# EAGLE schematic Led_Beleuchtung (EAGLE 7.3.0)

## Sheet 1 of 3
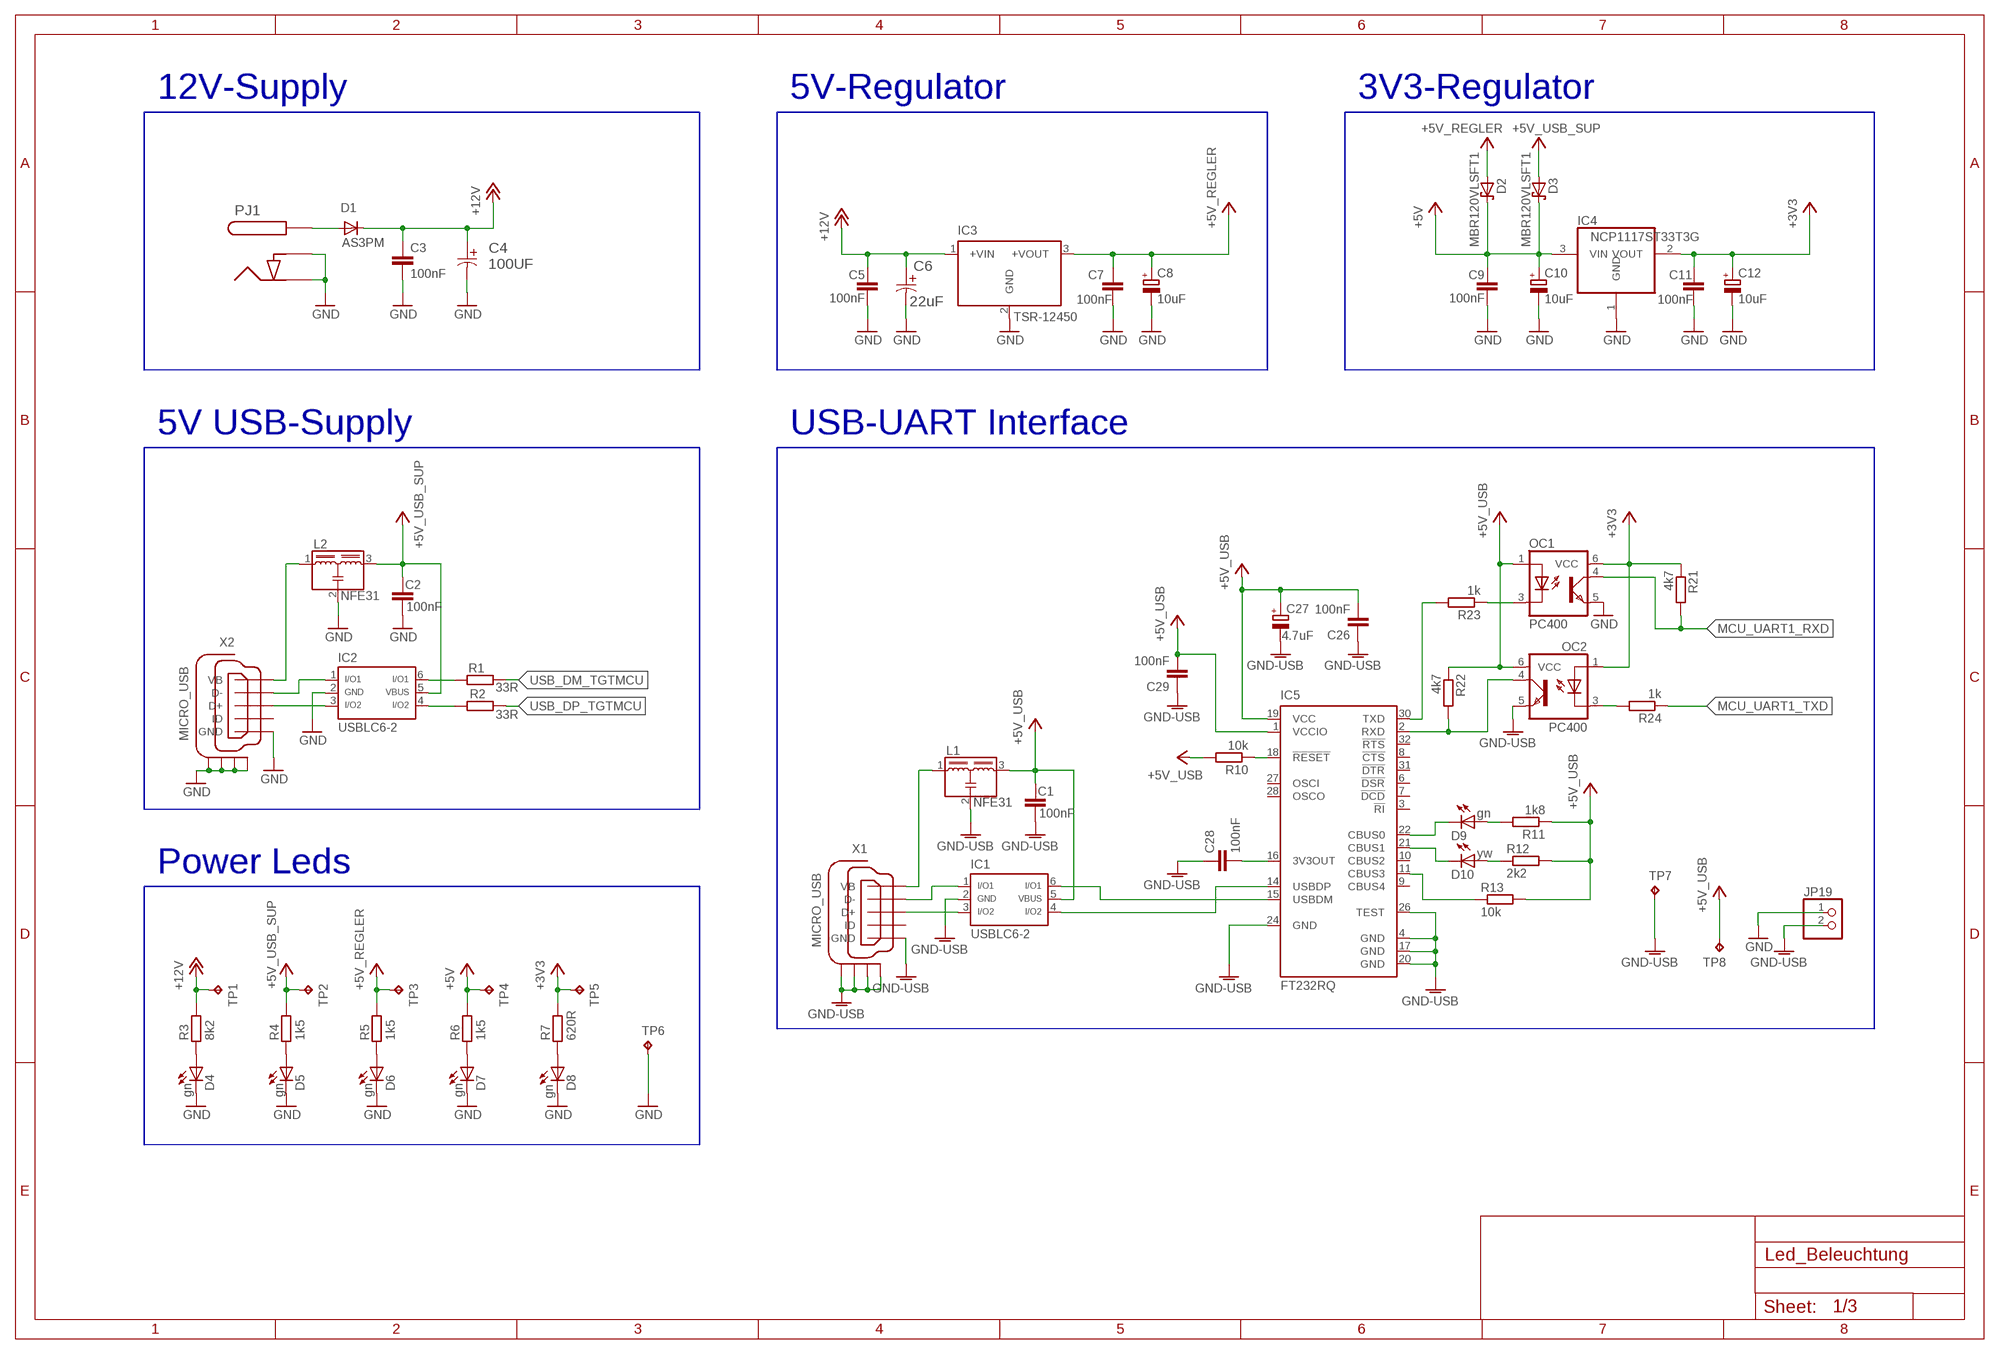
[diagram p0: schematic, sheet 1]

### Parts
C1  100nF  C-EUC0603K  [C0603K]
C2  100nF  C-EUC0603K  [C0603K]
C3  100nF  C-EUC0603K  [C0603K]
C4  100UF  EEE-FTH101XAP-CASE-D8  [CAPAE660X800N]
C5  100nF  C-EUC0603K  [C0603K]
C6  22uF  EEE--CASE-D  [CAPAE660X610N]
C7  100nF  C-EUC0603K  [C0603K]
C8  10uF  CPOL_EU0805  [SMC_P]
C9  100nF  C-EUC0603K  [C0603K]
C10  10uF  CPOL_EU0805  [SMC_P]
C11  100nF  C-EUC0603K  [C0603K]
C12  10uF  CPOL_EU0805  [SMC_P]
C26  100nF  C-EUC0603K  [C0603K]
C27  4.7uF  CPOL_EU0805  [SMC_P]
C28  100nF  C-EUC0603K  [C0603K]
C29  100nF  C-EUC0603  [C0603]
D1  AS3PM  [TO-277A]
D2  MBR120VLSFT1  [SOD-123]
D3  MBR120VLSFT1  [SOD-123]
D4  gn  LEDCHIP-LED0603  [CHIP-LED0603]
D5  gn  LEDCHIP-LED0603  [CHIP-LED0603]
D6  gn  LEDCHIP-LED0603  [CHIP-LED0603]
D7  gn  LEDCHIP-LED0603  [CHIP-LED0603]
D8  gn  LEDCHIP-LED0603  [CHIP-LED0603]
D9  gn  LEDCHIP-LED0603  [CHIP-LED0603]
D10  yw  LEDCHIP-LED0603  [CHIP-LED0603]
IC1  USBLC6-2  [SOT-23-6L]
IC2  USBLC6-2  [SOT-23-6L]
IC3  TSR-12450  [TSR-1]
IC4  NCP1117ST33T3G  REG1117  [SOT223]
IC5  FT232RQ  [QFN32]
JP19  PINHD-1X2  [1X02]
L1  NFE31  EMIFIL  [EMIFILTER]
L2  NFE31  EMIFIL  [EMIFILTER]
OC1  PC400  [PC400]
OC2  PC400  [PC400]
PJ1  PJ-002AH-SMT-TR  [PJ-002AH-SMT-TR]
R1  33R  R-EU_R0603  [R0603]
R2  33R  R-EU_R0603  [R0603]
R3  8k2  R-EU_R0603  [R0603]
R4  1k5  R-EU_R0603  [R0603]
R5  1k5  R-EU_R0603  [R0603]
R6  1k5  R-EU_R0603  [R0603]
R7  620R  R-EU_R0603  [R0603]
R10  10k  R-EU_R0603  [R0603]
R11  1k8  R-EU_R0603  [R0603]
R12  2k2  R-EU_R0603  [R0603]
R13  10k  R-EU_R0603  [R0603]
R21  4k7  R-EU_R0603  [R0603]
R22  4k7  R-EU_R0603  [R0603]
R23  1k  R-EU_R0603  [R0603]
R24  1k  R-EU_R0603  [R0603]
TP1  +12V  TPTP08R  [TP08R]
TP2  +5V_USB  TPTP08R  [TP08R]
TP3  +5V_Reg  TPTP08R  [TP08R]
TP4  +5V  TPTP08R  [TP08R]
TP5  +3V3  TPTP08R  [TP08R]
TP6  GND  TPTP08R  [TP08R]
TP7  GND  TPTP08R  [TP08R]
TP8  +5V  TPTP08R  [TP08R]
X1  MICRO_USB  [MICRO-USB]
X2  MICRO_USB  [MICRO-USB]

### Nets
3V3OUT_FT232: C28.2 IC5.16(3V3OUT)
+3V3: C11.2 C12.+ IC4.2(VOUT) OC1.6(VCC) OC2.1(A) R7.2 R21.1 TP5.TP ; also sheet 2
+5V: C9.2 C10.+ D2.C D3.C IC4.3(VIN) R6.2 TP4.TP ; also sheet 2
+5V_REGLER: C7.2 C8.+ D2.A IC3.3(+VOUT) R5.2 TP3.TP
+5V_USB: C1.2 C26.2 C27.+ C29.2 IC1.5 IC5.1(VCCIO) IC5.19(VCC) L1.3 OC1.1(A) OC2.6(VCC) R10.2 R11.1 R12.2 R13.2 R22.1 TP8.TP
+5V_USB_SUP: C2.2 D3.A IC2.5 L2.3 R4.2 TP2.TP
+12V: C3.2 C4.1 C5.2 C6.1 D1.C IC3.1(+VIN) R3.2 TP1.TP ; also sheet 3
GND: C2.1 C3.1 C4.2 C5.1 C6.2 C7.1 C8.- C9.1 C10.- C11.1 C12.- D4.C D5.C D6.C D7.C D8.C IC2.2 IC3.2(GND) IC4.1(GND) JP19.1 L2.2 OC1.5(EMI) PJ1.2 PJ1.3 TP6.TP X2.5(GND) X2.GND1(S1) X2.GND2(S2) X2.GND3(S3) X2.GND4(S4) ; also sheet 2,3
GND-USB: C1.1 C26.1 C27.- C28.1 C29.1 IC1.2 IC5.4(GND) IC5.17(GND) IC5.20(GND) IC5.24(GND) IC5.26(TEST) JP19.2 L1.2 OC2.5(EMI) TP7.TP X1.5(GND) X1.GND1(S1) X1.GND2(S2) X1.GND3(S3) X1.GND4(S4)
MCU_UART1_RXD: OC1.4(COL) R21.2 ; also sheet 2
MCU_UART1_TXD: R24.1 ; also sheet 2
N$3: IC5.18(!RESET) R10.1
N$9: D9.C IC5.22(CBUS0)
N$13: L1.1 X1.1(VB)
N$14: IC1.1 X1.2(D-)
N$15: IC1.3 X1.3(D+)
N$16: D4.A R3.1
N$17: L2.1 X2.1(VB)
N$18: D5.A R4.1
N$19: D10.C IC5.21(CBUS1)
N$21: D10.A R12.1
N$22: D9.A R11.2
N$23: IC5.11(CBUS3) R13.1
N$26: IC2.1 X2.2(D-)
N$27: IC2.3 X2.3(D+)
N$48: IC2.4 R2.1
N$49: IC2.6 R1.1
N$61: D6.A R5.1
N$86: D1.A1(A) D1.A2(A) PJ1.1.1 PJ1.1.2
N$88: D7.A R6.1
N$90: D8.A R7.1
N$91: OC1.3(C) R23.1
N$93: OC2.3(C) R24.2
N$95: IC5.30(TXD) R23.2
N$97: IC5.2(RXD) OC2.4(COL) R22.2
USB_DM_FT232: IC1.6 IC5.15(USBDM)
USB_DM_TGTMCU: R1.2 ; also sheet 2
USB_DP_FT232: IC1.4 IC5.14(USBDP)
USB_DP_TGTMCU: R2.2 ; also sheet 2
Unconnected: IC5.3(!RI) IC5.6(!DSR) IC5.7(!DCD) IC5.8(!CTS) IC5.9(CBUS4) IC5.10(CBUS2) IC5.27(OSCI) IC5.28(OSCO) IC5.31(!DTR) IC5.32(!RTS) X1.4(ID) X2.4(ID)

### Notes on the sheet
- 12V-Supply | 5V-Regulator | 3V3-Regulator
- 5V USB-Supply | USB-UART Interface
- Power Leds
- http://www.molex.com/pdm_docs/sd/5031821853_sd.pdf 
  http://pinouts.ru/Memory/sdcard_pinout.shtml 
  http://www.interfacebus.com/Secure_Digital_Card_Pinout.html 
  https://en.wikipedia.org/wiki/Secure_Digital

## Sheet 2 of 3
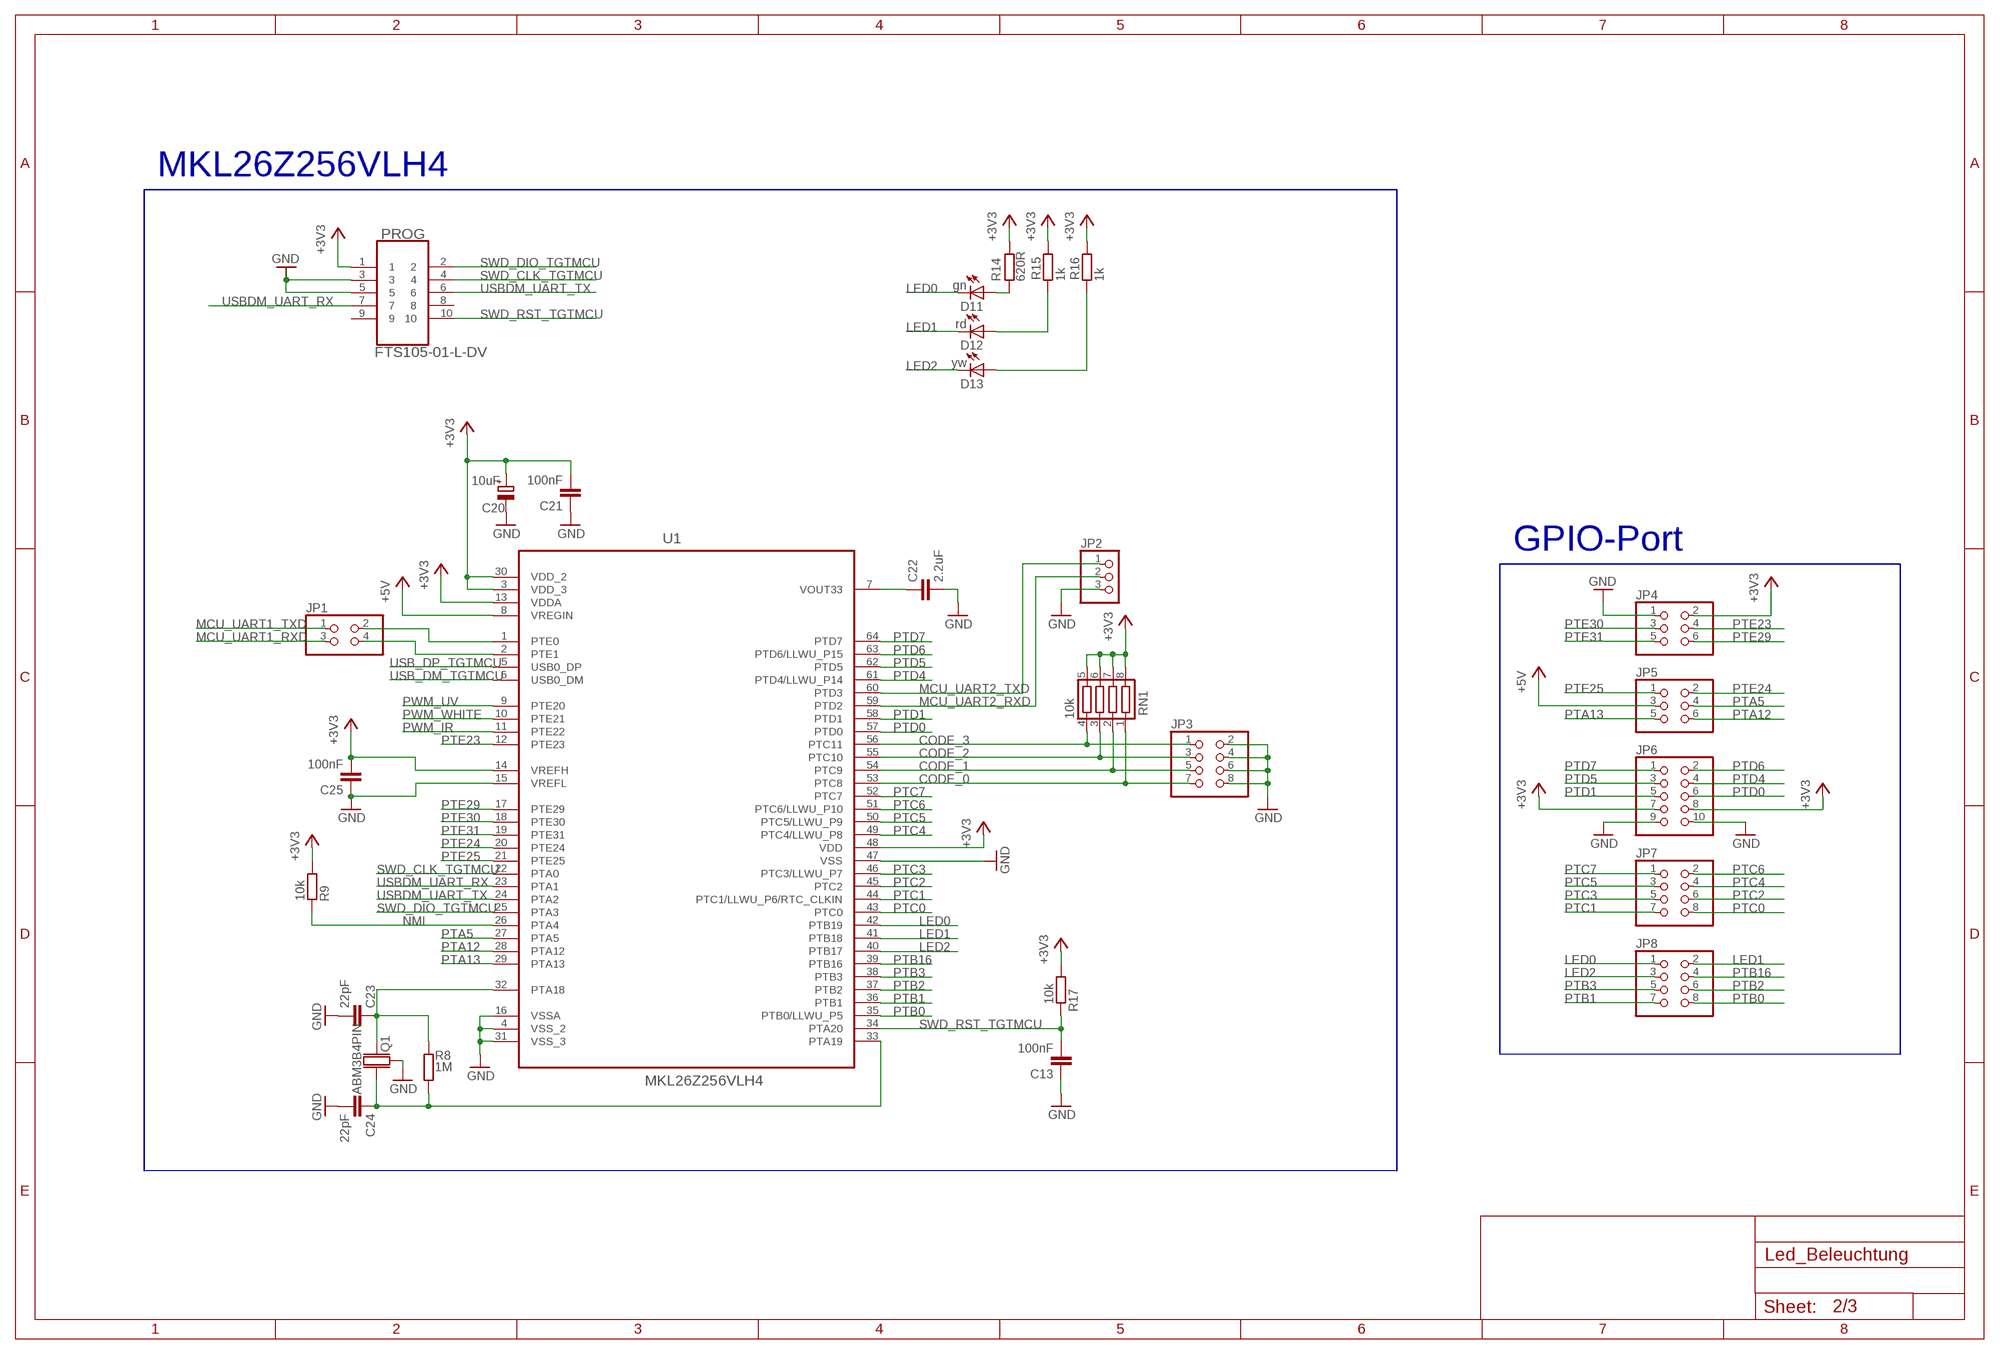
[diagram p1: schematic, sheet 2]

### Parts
C13  100nF  C-EUC0603  [C0603]
C20  10uF  CPOL_EU0805  [SMC_P]
C21  100nF  C-EUC0603  [C0603]
C22  2.2uF  C-EUC0603  [C0603]
C23  22pF  C-EUC0603  [C0603]
C24  22pF  C-EUC0603  [C0603]
C25  100nF  C-EUC0603K  [C0603K]
D11  gn  LEDCHIP-LED0603  [CHIP-LED0603]
D12  rd  LEDCHIP-LED0603  [CHIP-LED0603]
D13  yw  LEDCHIP-LED0603  [CHIP-LED0603]
JP1  PINHD-2X2  [2X02]
JP2  BCH-381H-3GN  [BCH-381H-3GN]
JP3  PINHD-2X4  [2X04]
JP4  PINHD-2X3  [2X03]
JP5  PINHD-2X3  [2X03]
JP6  PINHD-2X5  [2X05]
JP7  PINHD-2X4  [2X04]
JP8  PINHD-2X4  [2X04]
PROG  FTS105-01-L-DV  [SAMTEC_FTS105-01-L-DV]
Q1  ABM3B4PIN  [ABM3B]
R8  1M  R-EU_R0603  [R0603]
R9  10k  R-EU_R0603  [R0603]
R14  620R  R-EU_R0603  [R0603]
R15  1k  R-EU_R0603  [R0603]
R16  1k  R-EU_R0603  [R0603]
R17  10k  R-EU_R0603  [R0603]
RN1  10k  CTS742C083  [CTS742C083]
U1  MKL26Z256VLH4  [QFP50P1200X1200X160-64N]

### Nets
+3V3: C20.+ C21.2 C25.2 JP4.2 JP6.7 JP6.8 PROG.1 R9.1 R14.2 R15.2 R16.2 R17.1 RN1.5 RN1.6 RN1.7 RN1.8 U1.3(VDD_3) U1.13(VDDA) U1.14(VREFH) U1.30(VDD_2) U1.48(VDD) ; also sheet 1
+5V: JP5.3 U1.8(VREGIN) ; also sheet 1
CODE_0: JP3.7 RN1.1 U1.53(PTC8)
CODE_1: JP3.5 RN1.2 U1.54(PTC9)
CODE_2: JP3.3 RN1.3 U1.55(PTC10)
CODE_3: JP3.1 RN1.4 U1.56(PTC11)
GND: C13.1 C20.- C21.1 C22.2 C23.2 C24.2 C25.1 JP2.3 JP3.2 JP3.4 JP3.6 JP3.8 JP4.1 JP6.9 JP6.10 PROG.3 PROG.5 Q1.GND1(GND) Q1.GND2(GND) U1.4(VSS_2) U1.15(VREFL) U1.16(VSSA) U1.31(VSS_3) U1.47(VSS) ; also sheet 1,3
LED0: D11.C JP8.1 U1.42(PTB19)
LED1: D12.C JP8.2 U1.41(PTB18)
LED2: D13.C JP8.3 U1.40(PTB17)
MCU_UART1_RXD: JP1.3 ; also sheet 1
MCU_UART1_TXD: JP1.1 ; also sheet 1
MCU_UART2_RXD: JP2.2 U1.59(PTD2)
MCU_UART2_TXD: JP2.1 U1.60(PTD3)
N$10: C23.1 Q1.1 R8.2 U1.32(PTA18)
N$11: C24.1 Q1.3 R8.1 U1.33(PTA19)
N$12: D11.A R14.1
N$36: D12.A R15.1
N$37: D13.A R16.1
N$47: C22.1 U1.7(VOUT33)
N$92: JP1.2 U1.1(PTE0)
N$94: JP1.4 U1.2(PTE1)
NMI: R9.2 U1.26(PTA4)
PTA5: JP5.4 U1.27(PTA5)
PTA12: JP5.6 U1.28(PTA12)
PTA13: JP5.5 U1.29(PTA13)
PTB0: JP8.8 U1.35(PTB0/LLWU_P5)
PTB1: JP8.7 U1.36(PTB1)
PTB2: JP8.6 U1.37(PTB2)
PTB3: JP8.5 U1.38(PTB3)
PTB16: JP8.4 U1.39(PTB16)
PTC0: JP7.8 U1.43(PTC0)
PTC1: JP7.7 U1.44(PTC1/LLWU_P6/RTC_CLKIN)
PTC2: JP7.6 U1.45(PTC2)
PTC3: JP7.5 U1.46(PTC3/LLWU_P7)
PTC4: JP7.4 U1.49(PTC4/LLWU_P8)
PTC5: JP7.3 U1.50(PTC5/LLWU_P9)
PTC6: JP7.2 U1.51(PTC6/LLWU_P10)
PTC7: JP7.1 U1.52(PTC7)
PTD0: JP6.6 U1.57(PTD0)
PTD1: JP6.5 U1.58(PTD1)
PTD4: JP6.4 U1.61(PTD4/LLWU_P14)
PTD5: JP6.3 U1.62(PTD5)
PTD6: JP6.2 U1.63(PTD6/LLWU_P15)
PTD7: JP6.1 U1.64(PTD7)
PTE23: JP4.4 U1.12(PTE23)
PTE24: JP5.2 U1.20(PTE24)
PTE25: JP5.1 U1.21(PTE25)
PTE29: JP4.6 U1.17(PTE29)
PTE30: JP4.3 U1.18(PTE30)
PTE31: JP4.5 U1.19(PTE31)
PWM_IR: U1.11(PTE22) ; also sheet 3
PWM_UV: U1.9(PTE20) ; also sheet 3
PWM_WHITE: U1.10(PTE21) ; also sheet 3
SWD_CLK_TGTMCU: PROG.4 U1.22(PTA0)
SWD_DIO_TGTMCU: PROG.2 U1.25(PTA3)
SWD_RST_TGTMCU: C13.2 PROG.10 R17.2 U1.34(PTA20)
USB_DM_TGTMCU: U1.6(USB0_DM) ; also sheet 1
USB_DP_TGTMCU: U1.5(USB0_DP) ; also sheet 1
USBDM_UART_RX: PROG.7 U1.23(PTA1)
USBDM_UART_TX: PROG.6 U1.24(PTA2)
Unconnected: PROG.8 PROG.9

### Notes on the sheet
- MKL26Z256VLH4
- GPIO-Port

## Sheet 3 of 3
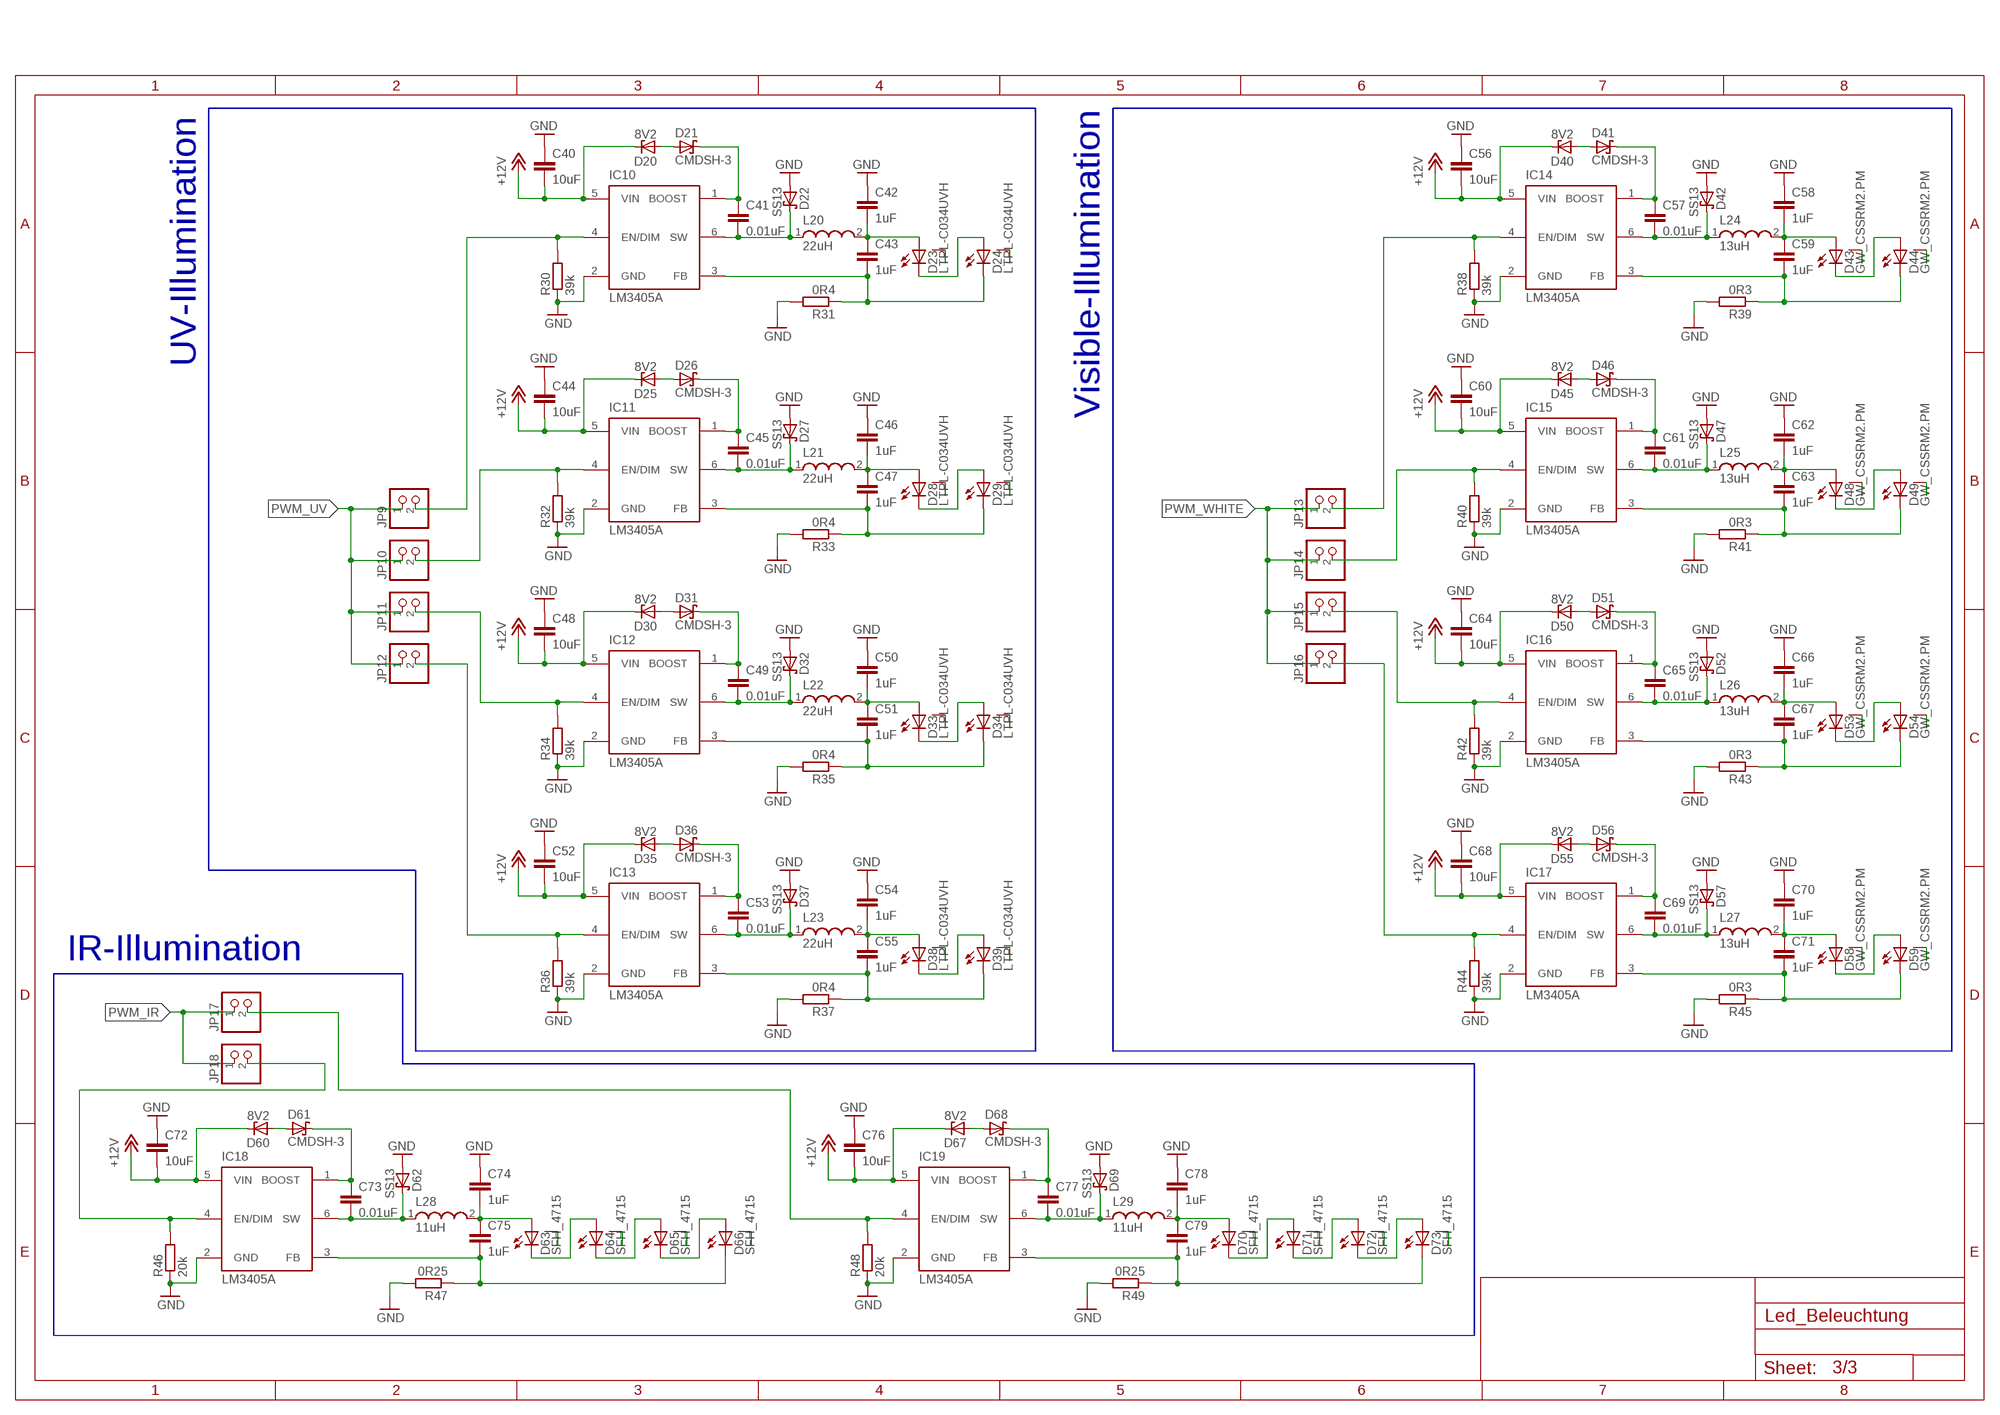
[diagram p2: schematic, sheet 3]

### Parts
C40  10uF  C-EUC1206K  [C1206K]
C41  0.01uF  C-EUC0805K  [C0805K]
C42  1uF  C-EUC1206K  [C1206K]
C43  1uF  C-EUC1206K  [C1206K]
C44  10uF  C-EUC1206K  [C1206K]
C45  0.01uF  C-EUC0805K  [C0805K]
C46  1uF  C-EUC1206K  [C1206K]
C47  1uF  C-EUC1206K  [C1206K]
C48  10uF  C-EUC1206K  [C1206K]
C49  0.01uF  C-EUC0805K  [C0805K]
C50  1uF  C-EUC1206K  [C1206K]
C51  1uF  C-EUC1206K  [C1206K]
C52  10uF  C-EUC1206K  [C1206K]
C53  0.01uF  C-EUC0805K  [C0805K]
C54  1uF  C-EUC1206K  [C1206K]
C55  1uF  C-EUC1206K  [C1206K]
C56  10uF  C-EUC1206K  [C1206K]
C57  0.01uF  C-EUC0805K  [C0805K]
C58  1uF  C-EUC1206K  [C1206K]
C59  1uF  C-EUC1206K  [C1206K]
C60  10uF  C-EUC1206K  [C1206K]
C61  0.01uF  C-EUC0805K  [C0805K]
C62  1uF  C-EUC1206K  [C1206K]
C63  1uF  C-EUC1206K  [C1206K]
C64  10uF  C-EUC1206K  [C1206K]
C65  0.01uF  C-EUC0805K  [C0805K]
C66  1uF  C-EUC1206K  [C1206K]
C67  1uF  C-EUC1206K  [C1206K]
C68  10uF  C-EUC1206K  [C1206K]
C69  0.01uF  C-EUC0805K  [C0805K]
C70  1uF  C-EUC1206K  [C1206K]
C71  1uF  C-EUC1206K  [C1206K]
C72  10uF  C-EUC1206K  [C1206K]
C73  0.01uF  C-EUC0805K  [C0805K]
C74  1uF  C-EUC1206K  [C1206K]
C75  1uF  C-EUC1206K  [C1206K]
C76  10uF  C-EUC1206K  [C1206K]
C77  0.01uF  C-EUC0805K  [C0805K]
C78  1uF  C-EUC1206K  [C1206K]
C79  1uF  C-EUC1206K  [C1206K]
D20  8V2  ZENER-DIODESOT23  [SOT23]
D21  CMDSH-3  [SOD323]
D22  SS13  [DO-214AC]
D23  LTPL-C034UVH  [LTPL-C034UVH]
D24  LTPL-C034UVH  [LTPL-C034UVH]
D25  8V2  ZENER-DIODESOT23  [SOT23]
D26  CMDSH-3  [SOD323]
D27  SS13  [DO-214AC]
D28  LTPL-C034UVH  [LTPL-C034UVH]
D29  LTPL-C034UVH  [LTPL-C034UVH]
D30  8V2  ZENER-DIODESOT23  [SOT23]
D31  CMDSH-3  [SOD323]
D32  SS13  [DO-214AC]
D33  LTPL-C034UVH  [LTPL-C034UVH]
D34  LTPL-C034UVH  [LTPL-C034UVH]
D35  8V2  ZENER-DIODESOT23  [SOT23]
D36  CMDSH-3  [SOD323]
D37  SS13  [DO-214AC]
D38  LTPL-C034UVH  [LTPL-C034UVH]
D39  LTPL-C034UVH  [LTPL-C034UVH]
D40  8V2  ZENER-DIODESOT23  [SOT23]
D41  CMDSH-3  [SOD323]
D42  SS13  [DO-214AC]
D43  GW_CSSRM2.PM  [GW_CSSRM2.PM]
D44  GW_CSSRM2.PM  [GW_CSSRM2.PM]
D45  8V2  ZENER-DIODESOT23  [SOT23]
D46  CMDSH-3  [SOD323]
D47  SS13  [DO-214AC]
D48  GW_CSSRM2.PM  [GW_CSSRM2.PM]
D49  GW_CSSRM2.PM  [GW_CSSRM2.PM]
D50  8V2  ZENER-DIODESOT23  [SOT23]
D51  CMDSH-3  [SOD323]
D52  SS13  [DO-214AC]
D53  GW_CSSRM2.PM  [GW_CSSRM2.PM]
D54  GW_CSSRM2.PM  [GW_CSSRM2.PM]
D55  8V2  ZENER-DIODESOT23  [SOT23]
D56  CMDSH-3  [SOD323]
D57  SS13  [DO-214AC]
D58  GW_CSSRM2.PM  [GW_CSSRM2.PM]
D59  GW_CSSRM2.PM  [GW_CSSRM2.PM]
D60  8V2  ZENER-DIODESOT23  [SOT23]
D61  CMDSH-3  [SOD323]
D62  SS13  [DO-214AC]
D63  SFH_4715  [SFH_4715]
D64  SFH_4715  [SFH_4715]
D65  SFH_4715  [SFH_4715]
D66  SFH_4715  [SFH_4715]
D67  8V2  ZENER-DIODESOT23  [SOT23]
D68  CMDSH-3  [SOD323]
D69  SS13  [DO-214AC]
D70  SFH_4715  [SFH_4715]
D71  SFH_4715  [SFH_4715]
D72  SFH_4715  [SFH_4715]
D73  SFH_4715  [SFH_4715]
IC10  LM3405A  [DDC6_SOT]
IC11  LM3405A  [DDC6_SOT]
IC12  LM3405A  [DDC6_SOT]
IC13  LM3405A  [DDC6_SOT]
IC14  LM3405A  [DDC6_SOT]
IC15  LM3405A  [DDC6_SOT]
IC16  LM3405A  [DDC6_SOT]
IC17  LM3405A  [DDC6_SOT]
IC18  LM3405A  [DDC6_SOT]
IC19  LM3405A  [DDC6_SOT]
JP9  PINHD-1X2  [1X02]
JP10  PINHD-1X2  [1X02]
JP11  PINHD-1X2  [1X02]
JP12  PINHD-1X2  [1X02]
JP13  PINHD-1X2  [1X02]
JP14  PINHD-1X2  [1X02]
JP15  PINHD-1X2  [1X02]
JP16  PINHD-1X2  [1X02]
JP17  PINHD-1X2  [1X02]
JP18  PINHD-1X2  [1X02]
L20  22uH  WE-PDF_1064  [WE-PDF]
L21  22uH  WE-PDF_1064  [WE-PDF]
L22  22uH  WE-PDF_1064  [WE-PDF]
L23  22uH  WE-PDF_1064  [WE-PDF]
L24  13uH  WE-PDF_1064  [WE-PDF]
L25  13uH  WE-PDF_1064  [WE-PDF]
L26  13uH  WE-PDF_1064  [WE-PDF]
L27  13uH  WE-PDF_1064  [WE-PDF]
L28  11uH  WE-PDF_1064  [WE-PDF]
L29  11uH  WE-PDF_1064  [WE-PDF]
R30  39k  R-EU_R0603  [R0603]
R31  0R4  R-EU_R2010  [R2010]
R32  39k  R-EU_R0603  [R0603]
R33  0R4  R-EU_R2010  [R2010]
R34  39k  R-EU_R0603  [R0603]
R35  0R4  R-EU_R2010  [R2010]
R36  39k  R-EU_R0603  [R0603]
R37  0R4  R-EU_R2010  [R2010]
R38  39k  R-EU_R0603  [R0603]
R39  0R3  R-EU_R2010  [R2010]
R40  39k  R-EU_R0603  [R0603]
R41  0R3  R-EU_R2010  [R2010]
R42  39k  R-EU_R0603  [R0603]
R43  0R3  R-EU_R2010  [R2010]
R44  39k  R-EU_R0603  [R0603]
R45  0R3  R-EU_R2010  [R2010]
R46  20k  R-EU_R0603  [R0603]
R47  0R25  R-EU_R2010  [R2010]
R48  20k  R-EU_R0603  [R0603]
R49  0R25  R-EU_R2010  [R2010]

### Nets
+12V: C40.2 C44.2 C48.2 C52.2 C56.2 C60.2 C64.2 C68.2 C72.2 C76.2 D20.3(C) D25.3(C) D30.3(C) D35.3(C) D40.3(C) D45.3(C) D50.3(C) D55.3(C) D60.3(C) D67.3(C) IC10.5(VIN) IC11.5(VIN) IC12.5(VIN) IC13.5(VIN) IC14.5(VIN) IC15.5(VIN) IC16.5(VIN) IC17.5(VIN) IC18.5(VIN) IC19.5(VIN) ; also sheet 1
GND: C40.1 C42.1 C44.1 C46.1 C48.1 C50.1 C52.1 C54.1 C56.1 C58.1 C60.1 C62.1 C64.1 C66.1 C68.1 C70.1 C72.1 C74.1 C76.1 C78.1 D22.A D27.A D32.A D37.A D42.A D47.A D52.A D57.A D62.A D69.A IC10.2(GND) IC11.2(GND) IC12.2(GND) IC13.2(GND) IC14.2(GND) IC15.2(GND) IC16.2(GND) IC17.2(GND) IC18.2(GND) IC19.2(GND) R30.1 R31.2 R32.1 R33.2 R34.1 R35.2 R36.1 R37.2 R38.1 R39.2 R40.1 R41.2 R42.1 R43.2 R44.1 R45.2 R46.1 R47.2 R48.1 R49.2 ; also sheet 1,2
LED_WHITE8: D58.C D59.A
N$1: C77.1 D68.C IC19.1(BOOST)
N$2: D67.1(A) D68.A
N$4: C77.2 D69.C IC19.6(SW) L29.1
N$5: C78.2 C79.1 D70.A L29.2
N$6: D70.C D71.A
N$7: D71.C D72.A
N$8: D72.C D73.A
N$20: C79.2 D73.C IC19.3(FB) R49.1
N$24: C57.1 D41.C IC14.1(BOOST)
N$25: C73.1 D61.C IC18.1(BOOST)
N$28: D60.1(A) D61.A
N$29: C73.2 D62.C IC18.6(SW) L28.1
N$30: C74.2 C75.1 D63.A L28.2
N$31: D63.C D64.A
N$32: D64.C D65.A
N$33: D65.C D66.A
N$34: C75.2 D66.C IC18.3(FB) R47.1
N$35: D40.1(A) D41.A
N$38: C57.2 D42.C IC14.6(SW) L24.1
N$39: C58.2 C59.1 D43.A L24.2
N$40: D43.C D44.A
N$41: C61.1 D46.C IC15.1(BOOST)
N$42: D45.1(A) D46.A
N$43: C59.2 D44.C IC14.3(FB) R39.1
N$44: C61.2 D47.C IC15.6(SW) L25.1
N$45: C62.2 C63.1 D48.A L25.2
N$46: D48.C D49.A
N$50: C63.2 D49.C IC15.3(FB) R41.1
N$51: C65.1 D51.C IC16.1(BOOST)
N$52: D50.1(A) D51.A
N$53: C65.2 D52.C IC16.6(SW) L26.1
N$54: C66.2 C67.1 D53.A L26.2
N$55: D53.C D54.A
N$56: C67.2 D54.C IC16.3(FB) R43.1
N$57: C69.1 D56.C IC17.1(BOOST)
N$58: D55.1(A) D56.A
N$59: C69.2 D57.C IC17.6(SW) L27.1
N$60: C70.2 C71.1 D58.A L27.2
N$62: C71.2 D59.C IC17.3(FB) R45.1
N$63: C41.1 D21.C IC10.1(BOOST)
N$64: D20.1(A) D21.A
N$65: C41.2 D22.C IC10.6(SW) L20.1
N$66: C42.2 C43.1 D23.A L20.2
N$67: D23.C D24.A
N$68: C43.2 D24.C IC10.3(FB) R31.1
N$69: C45.1 D26.C IC11.1(BOOST)
N$70: D25.1(A) D26.A
N$71: C45.2 D27.C IC11.6(SW) L21.1
N$72: C46.2 C47.1 D28.A L21.2
N$73: D28.C D29.A
N$74: C47.2 D29.C IC11.3(FB) R33.1
N$75: C49.1 D31.C IC12.1(BOOST)
N$76: D30.1(A) D31.A
N$77: C49.2 D32.C IC12.6(SW) L22.1
N$78: C50.2 C51.1 D33.A L22.2
N$79: D33.C D34.A
N$80: C51.2 D34.C IC12.3(FB) R35.1
N$81: C53.1 D36.C IC13.1(BOOST)
N$82: D35.1(A) D36.A
N$83: C53.2 D37.C IC13.6(SW) L23.1
N$84: C54.2 C55.1 D38.A L23.2
N$85: D38.C D39.A
N$87: C55.2 D39.C IC13.3(FB) R37.1
N$98: IC10.4(EN/DIM) JP9.2 R30.2
N$99: IC11.4(EN/DIM) JP10.2 R32.2
N$100: IC12.4(EN/DIM) JP11.2 R34.2
N$101: IC13.4(EN/DIM) JP12.2 R36.2
N$102: IC14.4(EN/DIM) JP13.2 R38.2
N$103: IC15.4(EN/DIM) JP14.2 R40.2
N$104: IC16.4(EN/DIM) JP15.2 R42.2
N$105: IC17.4(EN/DIM) JP16.2 R44.2
N$106: IC18.4(EN/DIM) JP18.2 R46.2
N$107: IC19.4(EN/DIM) JP17.2 R48.2
PWM_IR: JP17.1 JP18.1 ; also sheet 2
PWM_UV: JP9.1 JP10.1 JP11.1 JP12.1 ; also sheet 2
PWM_WHITE: JP13.1 JP14.1 JP15.1 JP16.1 ; also sheet 2
TH_D23: D23.TH
TH_D24: D24.TH
TH_D28: D28.TH
TH_D29: D29.TH
TH_D33: D33.TH
TH_D34: D34.TH
TH_D38: D38.TH
TH_D39: D39.TH
TH_D43: D43.TH
TH_D44: D44.TH
TH_D48: D48.TH
TH_D49: D49.TH
TH_D53: D53.TH
TH_D54: D54.TH
TH_D58: D58.TH
TH_D59: D59.TH
TH_D63: D63.TH
TH_D64: D64.TH
TH_D65: D65.TH
TH_D66: D66.TH
TH_D70: D70.TH
TH_D71: D71.TH
TH_D72: D72.TH
TH_D73: D73.TH

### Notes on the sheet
- UV-Illumination
- Visible-Illumination
- IR-Illumination

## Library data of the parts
C1-C3 C5 C7 C9 C11 C13 C21-C26 C28 C29 C40-C79 = rcl:C-EU: CAPACITOR, European symbol
C4 = Panasonic-EEEFT_EEEH:EEE-: Aluminum Electrolytic Capacitors,Surface Mount Type; MPN: EEE-FTH101XAP; OC_FARNELL: 1868426; OC_NEWARK: 31T8172; PACKAGE: CASE-D8; SUPPLIER: PANASONIC; TOLERANCE: ±20 %; VOLTAGERATING: 50V
C6 = Panasonic-EEEFT_EEEH:EEE-: Aluminum Electrolytic Capacitors,Surface Mount Type
C8 C10 C12 C20 C27 = myLib:CPOL_EU: Solid Tantalum SMD Cap, Size 0805 or P
D1 = myLib:AS3PM: http://www.mouser.com/ds/2/427/as3pd-101473.pdf
D2 D3 = myLib:MBR120VLSFT1: Schottky Power Rectifier
D4-D13 = led:LED: LED
D20 D25 D30 D35 D40 D45 D50 D55 D60 D67 = diode:ZENER-DIODE: Z-Diode
D21 D26 D31 D36 D41 D46 D51 D56 D61 D68 = myLib:CMDSH-3: http://www.mouser.com/ds/2/68/cmdsh-3-39175.pdf
D22 D27 D32 D37 D42 D47 D52 D57 D62 D69 = myLib:SS13: http://www.mouser.com/ds/2/427/ss12-100300.pdf
D23 D24 D28 D29 D33 D34 D38 D39 = myLib:LTPL-C034UVH: LITEON Led High Power LTPL-C034UVH385 Source: http://www.mouser.com/ds/2/239/LTPL-C034UVH385%20DataSheet_Ver4_20150916-775666.pdf
D43 D44 D48 D49 D53 D54 D58 D59 = myLib:GW_CSSRM2.PM: OSLON ® Square: GW CSSRM2.PM Source: http://www.mouser.com/ds/2/311/GW%20CSSRM2.PM%20-%20OSLON%20Square%20Gen%203%20(EnglishDeutsch)-1073956.pdf
D63-D66 D70-D73 = myLib:SFH_4715: OSLON Black Series (850 nm) - 90° SFH 4715 Source: http://www.osram-os.com/Graphics/XPic7/00204173_0.pdf
IC1 IC2 = myLib:USBLC6-2: http://www.farnell.com/datasheets/1690354.pdf?_ga=1.240650499.1400796248.1488872329
IC3 = myLib:TSR-1: DC/DC Converter TSR-1 Series Source: http://www.farnell.com/datasheets/1763604.pdf?_ga=1.177088805.1400796248.1488872329
IC4 = burr-brown:REG1117: 800mA and 1A Low Dropout (LDO) Positive Regulator 1.8V, 2.5V, 2.85V, 3.3V, 5V, and Adj; MPN: REG1117; OC_FARNELL: 1097566; OC_NEWARK: 14P6981
IC5 = ftdichip:FT232R: Source: http://www.ftdichip.com/Documents/DataSheets/DS_FT232R_v104.pdf; MPN: FT232RQ; OC_FARNELL: 1146033; OC_NEWARK: 91K9919
IC10-IC19 = myLib:LM3405A: 1-A Constant Current Buck LED Driver With Internal Compensation APPLICATIONS: LED Drivers Constant Current Sources Industrial Lighting LED Flashlights LED Lightbulbs Source: http://www.ti.com/lit/ds/symlink/lm3405a.pdf
JP1 = pinhead:PINHD-2X2: PIN HEADER
JP2 = myLib:BCH-381H-3GN: Printed-circuit board connectorR http://www.mouser.com/ds/2/324/ItemDetail_5444275-932016.pdf
JP3 JP7 JP8 = pinhead:PINHD-2X4: PIN HEADER
JP4 JP5 = pinhead:PINHD-2X3: PIN HEADER
JP6 = pinhead:PINHD-2X5: PIN HEADER
JP9-JP19 = pinhead:PINHD-1X2: PIN HEADER
L1 L2 = myLib:EMIFIL
L20-L29 = EAGLE-POWER_MAGNETICS-rev17a:WE-PDF: SMD Shielded Flatwire Power Inductor
OC1 OC2 = myLib:PC400: Source: http://www.mouser.com/ds/2/365/pc400_e-184091.pdf
PJ1 = power_jack:PJ-002AH-SMT-TR
PROG = myLib:FTS105-01-L-DV
Q1 = myLib:ABM3B: Quarz 8 MHz: http://www.abracon.com/Resonators/abm3b.pdf
R1-R17 R21-R24 R30-R49 = rcl:R-EU_: RESISTOR, European symbol
RN1 = resistor-net:CTS742C083: Chip Resistor Array 4 Single Resistor Source: http://www.ctscorp.com/components/Datasheets/CTSChipArrayDs.pdf; OC_FARNELL: unknown; OC_NEWARK: unknown
TP1-TP8 = testpad:TP: Test pad
U1 = myLib:MKL26Z256VLH4: 16BIT MCU, CORTEX M0+, 48MHZ, 64QFP; MPN: MKL26Z256VLH4; OC_FARNELL: 2360680; OC_NEWARK: 09X0214; PACKAGE: LQFP-64; SUPPLIER: FREESCALE SEMICONDUCTOR
X1 X2 = myLib:MICRO_USB: http://www.farnell.com/datasheets/1469072.pdf?_ga=1.139799603.1400796248.1488872329

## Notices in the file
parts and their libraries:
EAGLE-POWER_MAGNETICS-rev17a: Copyright: Würth Elektronik
